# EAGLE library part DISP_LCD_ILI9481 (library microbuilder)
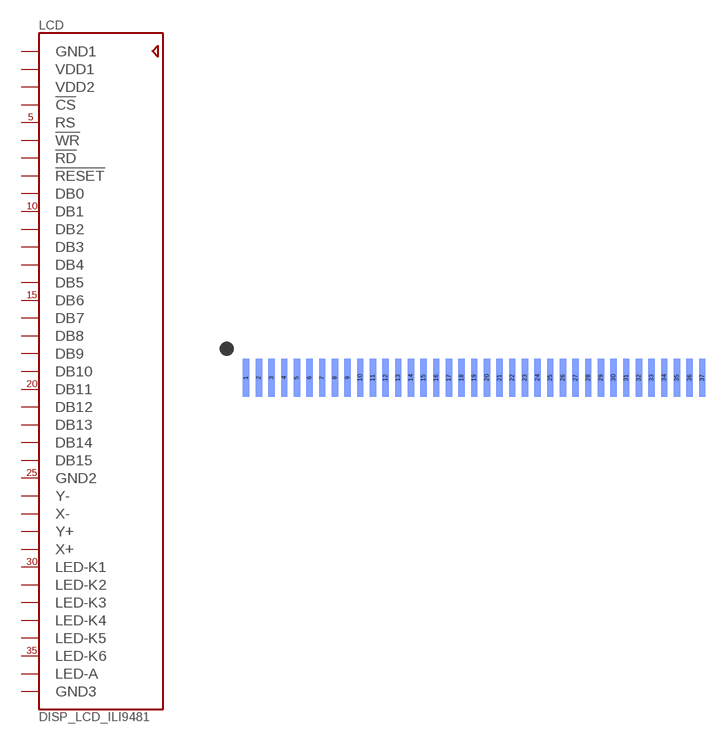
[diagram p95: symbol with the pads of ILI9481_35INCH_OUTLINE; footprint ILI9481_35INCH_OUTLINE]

Designator prefix LCD

## DISP_LCD_ILI9481  [ILI9481_35INCH_OUTLINE]
1  GND1  pas
2  VDD1  pas
3  VDD2  pas
4  !CS  pas
5  RS  pwr
6  !WR  pwr
7  !RD  pas
8  !RESET  pas
9  DB0  pas
10  DB1  pas
11  DB2  pas
12  DB3  pas
13  DB4  pas
14  DB5  pas
15  DB6  pas
16  DB7  pas
17  DB8  pas
18  DB9  pas
19  DB10  pas
20  DB11  pas
21  DB12  pas
22  DB13  pas
23  DB14  pas
24  DB15  pas
25  GND2  pas
26  Y-  pas
27  X-  pas
28  Y+  pas
29  X+  pas
30  LED-K1  pas
31  LED-K2  pas
32  LED-K3  pwr
33  LED-K4  pwr
34  LED-K5  pwr
35  LED-K6  pas
36  LED-A  pas
37  GND3  pas

## Footprint ILI9481_35INCH_OUTLINE (pad centres in mm)
smd 0.5 x 3 bottom: 1 -18,48.57; 2 -17,48.57; 3 -16,48.57; 4 -15,48.57; 5 -14,48.57; 6 -13,48.57; 7 -12,48.57; 8 -11,48.57; 9 -10,48.57; 10 -9,48.57; 11 -8,48.57; 12 -7,48.57; 13 -6,48.57; 14 -5,48.57; 15 -4,48.57; 16 -3,48.57; 17 -2,48.57; 18 -1,48.57; 19 0,48.57; 20 1,48.57; 21 2,48.57; 22 3,48.57; 23 4,48.57; 24 5,48.57; 25 6,48.57; 26 7,48.57; 27 8,48.57; 28 9,48.57; 29 10,48.57; 30 11,48.57; 31 12,48.57; 32 13,48.57; 33 14,48.57; 34 15,48.57; 35 16,48.57; 36 17,48.57; 37 18,48.57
